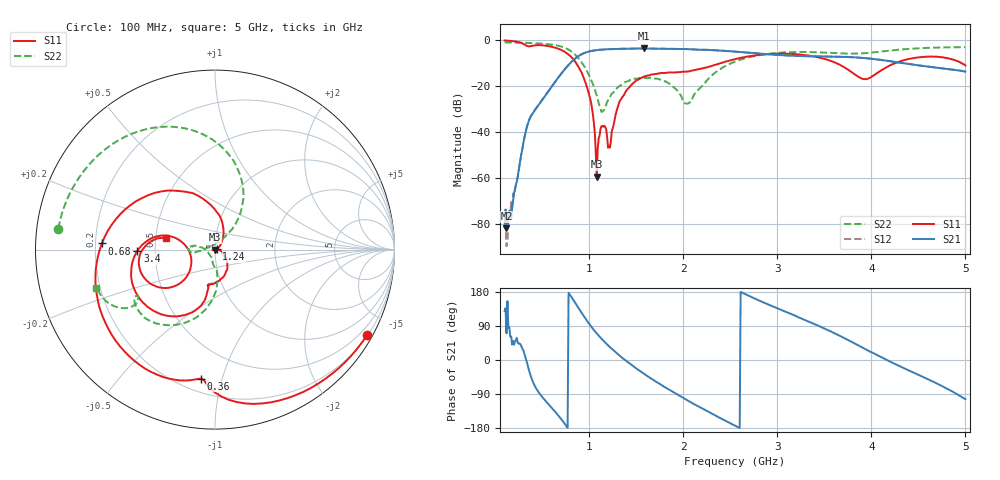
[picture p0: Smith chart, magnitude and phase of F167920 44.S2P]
!  2-Port S-parameters saved by WinCal
! VAR MeasName=S-Parameters (CALIBRATED_DATA) read from VNA (N5242A)
! VAR MeasDate=2016-11-22 9:57:40
! VAR NAME=F167920 44
! VAR FILENAME=F167920 44.S2P
! VAR DATE=2016-11-22 9:57:40
! VAR PHYS_PORTS=1,2
# Hz S DB R 50
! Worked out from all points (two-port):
!   491 points, 100 MHz to 5 GHz, reference 50 ohm
!   highest |S21| = -3.74 dB at 1.58 GHz (marker M1); lowest = -82.0 dB at 120 MHz (marker M2)
!   |S21| within 3 dB of the highest: 898 MHz to 3.086 GHz (2.188 GHz wide, 110 % of centre)
!   lowest |S11| = -59.6 dB at 1.08 GHz (marker M3), VSWR 1.00, Z = 49.9 - j0.053 ohm
!   |S11| at or under -10 dB: 859.1 MHz to 2.409 GHz (1.549 GHz wide, 94.8 % of centre); 3.621 GHz to 4.261 GHz (639.7 MHz wide, 16.2 % of centre); 4.955 GHz to end of sweep
!   |S22| runs from -31.3 to -1.1 dB; largest |S21 - S12| = 0.0012
!   S11 on the Smith chart (normalised r, x): 100 MHz: 0.22, -3.82; 360 MHz: 0.28, -0.85; 680 MHz: 0.23, +0.03; 1.24 GHz: 1.02, +0.01; 3.4 GHz: 0.40, -0.01; 5 GHz: 0.57, +0.08
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1e8  -0.25 -29.3  -81.45 129.3  -74.81 107.6  -1.10 172.4
1.2e8  -0.30 -35.0  -82.01 70.2  -89.79 70.3  -1.11 170.8
1.9e8  -0.56 -55.2  -70.17 50.6  -66.91 54.2  -1.16 165.5
3.6e8  -2.82 -96.3  -34.97 -28.2  -34.91 -27.7  -1.36 151.3
6.8e8  -4.00 176.9  -15.89 -149.1  -15.88 -149.2  -2.65 111.6
8e8  -7.11 132.7  -10.01 170.2  -10.01 170.2  -4.74 87.0
9.2e8  -14.32 82.6  -6.21 124.2  -6.21 124.2  -9.84 60.7
1.02e9  -27.47 41.4  -4.83 88.5  -4.83 88.5  -17.47 50.5
1.08e9  -59.56 -149.7  -4.47 70.0  -4.47 70.0  -24.32 57.5
1.14e9  -37.47 -173.4  -4.21 53.5  -4.21 53.5  -31.24 119.7
1.21e9  -46.09 135.6  -4.05 36.1  -4.05 36.1  -25.83 174.4
1.24e9  -39.78 26.0  -3.99 29.5  -3.99 29.5  -23.36 -179.4
1.34e9  -25.70 -28.4  -3.88 8.0  -3.87 8.0  -19.59 -173.2
1.58e9  -16.02 -72.5  -3.74 -35.9  -3.75 -35.9  -16.62 179.1
1.74e9  -14.58 -90.7  -3.84 -61.7  -3.83 -61.7  -17.14 173.3
2.05e9  -13.75 -100.6  -4.03 -107.4  -4.03 -107.4  -27.72 -137.9
2.55e9  -8.37 -111.6  -5.10 -173.2  -5.09 -173.2  -9.46 -98.8
3.37e9  -7.05 -176.6  -7.16 97.6  -7.16 97.5  -5.31 -144.5
3.4e9  -7.29 -179.0  -7.19 94.3  -7.18 94.3  -5.35 -145.5
3.92e9  -17.07 -169.4  -7.89 30.8  -7.88 30.9  -5.82 -147.2
4.19e9  -11.27 -136.2  -9.23 -3.2  -9.22 -3.1  -4.68 -146.2
5e9  -11.08 166.5  -13.79 -103.4  -13.79 -103.4  -3.17 -162.0
